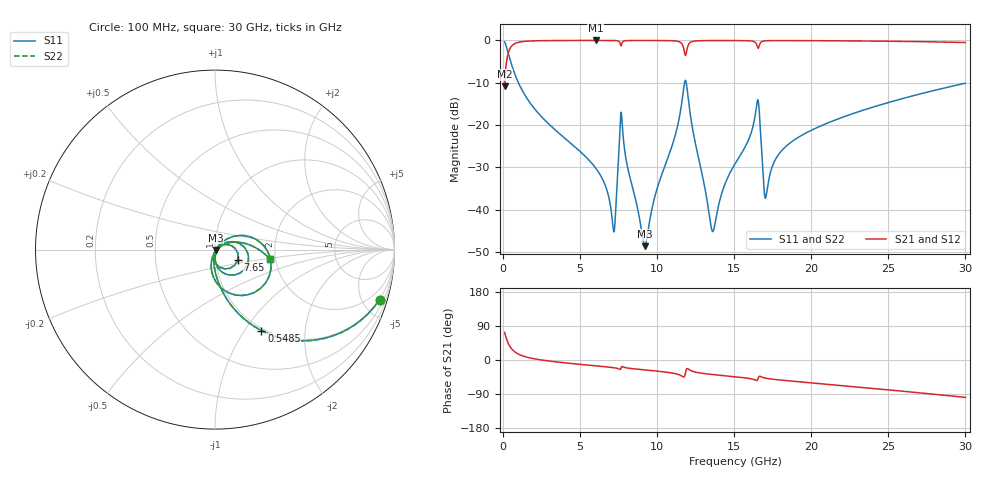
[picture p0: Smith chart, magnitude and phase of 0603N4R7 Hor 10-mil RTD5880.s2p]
# GHz S MA R 50
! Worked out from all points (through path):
!   3201 points, 100 MHz to 30 GHz, reference 50 ohm
!   highest |S21| = -0.03 dB at 6.024 GHz (marker M1); lowest = -10.9 dB at 100 MHz (marker M2)
!   group delay of S21, straight-line fit = 10.1 ps
!   lowest |S11| = -48.6 dB at 9.201 GHz (marker M3), VSWR 1.01, Z = 50.3 - j0.165 ohm
!   |S11| at or under -10 dB: 995.7 MHz to 11.78 GHz (10.78 GHz wide, 169 % of centre); 11.89 GHz to end of sweep
!   |S22| runs from -48.6 to -0.4 dB; largest |S21 - S12| = 0
!   S11 on the Smith chart (normalised r, x): 100 MHz: 0.97, -6.59; 548.5 MHz: 0.97, -1.20; 7.65 GHz: 1.29, -0.14; 30 GHz: 1.87, -0.22
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0.1  0.9582 -16.9  0.2859 73.1  0.2859 73.1  0.9582 -16.9
0.5485  0.5201 -60.2  0.8534 29.8  0.8534 29.8  0.5201 -60.2
1.538938  0.2083 -82.1  0.9769 7.6  0.9769 7.6  0.2083 -82.1
5.089563  0.04721 -99.1  0.9965 -11.9  0.9965 -11.9  0.04721 -99.1
6.023937  0.03087 -100.5  0.9968 -15.5  0.9968 -15.5  0.03087 -100.5
6.696688  0.01802 -97.7  0.9965 -18.1  0.9965 -18.1  0.01802 -97.7
7.173219  0.005624 -44.0  0.9947 -20.3  0.9947 -20.3  0.005624 -44.0
7.304031  0.00948 19.3  0.9927 -21.2  0.9927 -21.2  0.00948 19.3
7.64975  0.1397 -23.3  0.8603 -21.6  0.8603 -21.6  0.1397 -23.3
9.200812  0.003731 -26.0  0.9961 -26.2  0.9961 -26.2  0.003731 -26.0
10.06978  0.01967 46.8  0.9951 -29.7  0.9951 -29.7  0.01967 46.8
11.54609  0.1595 29.6  0.9363 -41.4  0.9363 -41.4  0.1595 29.6
11.82641  0.3376 -29.5  0.6635 -35.5  0.6635 -35.5  0.3376 -29.5
12.18147  0.1216 -98.7  0.9534 -27.8  0.9534 -27.8  0.1216 -98.7
13.56434  0.005653 -46.3  0.9942 -38.2  0.9942 -38.2  0.005653 -46.3
15.05  0.03485 37.0  0.9939 -44.2  0.9939 -44.2  0.03485 37.0
16.48894  0.1888 -10.4  0.8536 -53.5  0.8536 -53.5  0.1888 -10.4
17.04956  0.01404 -16.7  0.9877 -48.0  0.9877 -48.0  0.01404 -16.7
17.91853  0.04611 30.5  0.9931 -52.6  0.9931 -52.6  0.04611 30.5
20.03956  0.08755 26.1  0.9908 -60.5  0.9908 -60.5  0.08755 26.1
25.01978  0.1851 9.3  0.9764 -78.9  0.9764 -78.9  0.1851 9.3
30  0.3119 -9.9  0.9425 -98.6  0.9425 -98.6  0.3119 -9.9
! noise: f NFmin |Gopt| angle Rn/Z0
0.1  0.0003815  0.9376  0.69  0.001364
3.417  0.003679  0.7935  9.925  0.003651
6.743  0.006985  0.7872  19.28  0.006566
10.06  0.01  0.7809  28.53  0.008799
13.39  0.01307  0.7794  37.75  0.01089
16.7  0.0485  0.9209  46.71  0.1144
20.03  0.01473  0.7238  55.21  0.00837
23.35  0.01671  0.721  63.53  0.008665
26.67  0.019  0.7235  71.62  0.009089
30  0.02151  0.7287  79.46  0.009493
